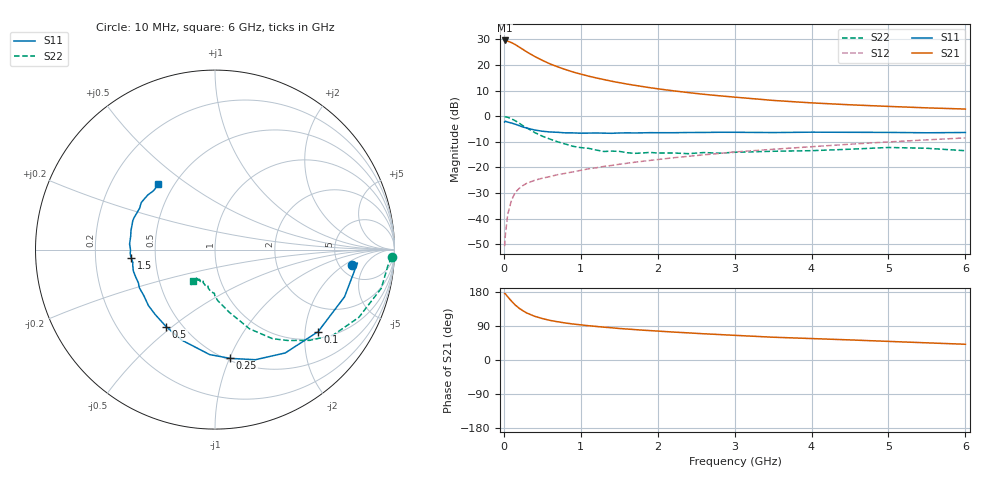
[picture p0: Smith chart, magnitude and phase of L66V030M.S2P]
!  INFINEON TECHNOLOGIES Small Signal Semiconductors
! BFR380L3 , Si-NPN RF-Transistor in TSLP-3-1
!  Vce=6 V,  Ic=30 mA
! Common Emitter S-Parameters:  07. March 2005
#  GHz  S  MA  R  50
! f  S11  S21  S12  S22
! GHz  Mag  Ang  Mag  Ang  Mag  Ang  Mag  Ang
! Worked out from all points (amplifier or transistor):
!   36 points, 10 MHz to 6 GHz, reference 50 ohm
!   highest |S21| = 29.6 dB at 10 MHz (marker M1)
!   |S21| within 3 dB of that: start of sweep to 221.9 MHz
!   unconditionally stable (mu >= 1): 2.222 GHz to 4.744 GHz
!   at 250 MHz: K = 0.35, MSG = 26.5 dB, |S12| = -27.0 dB
!   at 1.4 GHz: K = 0.93, MSG = 16.5 dB, |S12| = -19.2 dB
!   at 6 GHz: K = 0.97, MSG = 5.6 dB, |S12| = -8.5 dB
!   S11 on the Smith chart (normalised r, x): 10 MHz: 6.52, -2.75; 100 MHz: 1.18, -2.34; 250 MHz: 0.52, -1.01; 500 MHz: 0.41, -0.48; 1.5 GHz: 0.36, -0.04; 6 GHz: 0.41, +0.39
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0.01  0.7703 -6.4  30.09 175.3  0.0029 71.6  0.9862 -2.5
0.02  0.797 -5.4  29.81 174.7  0.0048 80.4  0.9675 -5.3
0.05  0.7682 -20.0  29.22 166.9  0.012 77.9  0.9512 -13.1
0.1  0.7342 -38.5  27.27 155.2  0.0231 72.0  0.8861 -25.2
0.15  0.6963 -55.8  24.9 144.8  0.0327 64.3  0.8121 -36.0
0.2  0.6533 -69.9  22.34 136.4  0.0391 62.3  0.7305 -43.8
0.25  0.612 -82.0  20.04 129.7  0.0445 56.6  0.6489 -51.3
0.3  0.5857 -92.9  17.92 123.9  0.0492 55.0  0.5903 -57.2
0.4  0.5376 -109.9  14.69 115.4  0.0559 52.6  0.4809 -66.5
0.5  0.5086 -122.3  12.31 109.4  0.0616 52.6  0.4072 -71.9
0.6  0.4918 -132.6  10.51 104.5  0.0662 52.5  0.3569 -77.3
0.7  0.4847 -139.9  9.188 100.9  0.0722 53.6  0.3157 -82.0
0.9  0.4721 -153.3  7.288 95.0  0.0819 55.5  0.2581 -90.1
1.1  0.4677 -161.3  6.057 90.5  0.0937 57.4  0.2359 -95.5
1.5  0.4699 -174.4  4.516 83.2  0.1151 60.2  0.2059 -105.5
1.8  0.4731 178.2  3.796 78.8  0.1315 61.1  0.1912 -111.0
2.2  0.4757 170.7  3.135 73.8  0.1541 62.0  0.1912 -115.3
2.8  0.4854 160.7  2.504 67.2  0.1873 62.9  0.1893 -123.0
3.5  0.4791 151.3  2.032 60.1  0.2258 61.7  0.2066 -123.7
4.5  0.4847 144.7  1.669 53.0  0.2838 61.0  0.2265 -124.6
5.5  0.4743 136.4  1.454 45.3  0.3449 58.1  0.2363 -124.7
6  0.4806 131.0  1.378 41.5  0.3768 56.1  0.2119 -125.5
